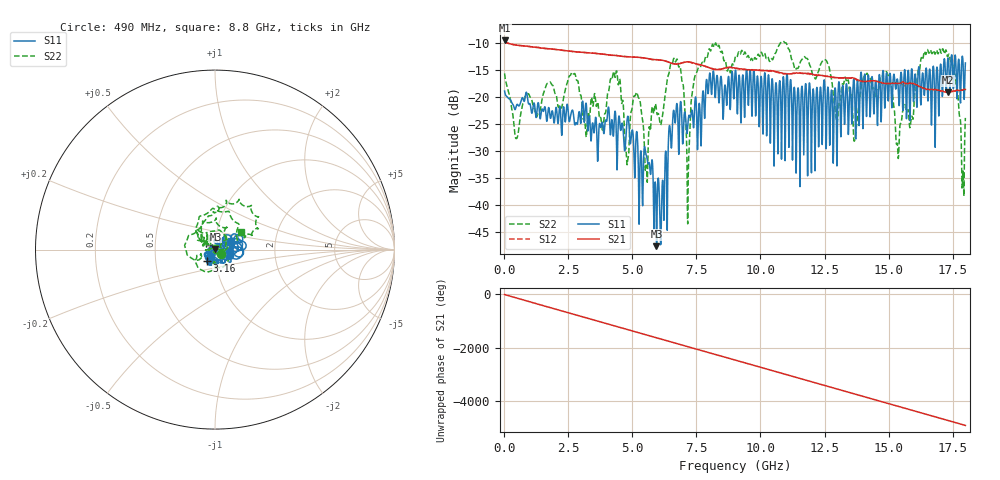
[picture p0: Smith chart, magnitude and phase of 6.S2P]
!Agilent Technologies,E5071C,MY46316741,A.11.02
!Date: Thu Sep 29 15:34:00 2022
!Data & Calibration Information:
!Freq	S11:SOLT2(ON)	S21:SOLT2(ON)	S12:SOLT2(ON)	S22:SOLT2(ON)
!PortZ  Port1:50+j0  Port2:50+j0
!Above PortZ is port z conversion or system Z0 setting when saving the data.
!When reading, reference impedance value at option line is always used.
# Hz S dB R 50
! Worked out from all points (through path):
!   1800 points, 10 MHz to 18 GHz, reference 50 ohm
!   highest |S21| = -9.45 dB at 10 MHz (marker M1); lowest = -19.0 dB at 17.31 GHz (marker M2)
!   group delay of S21, straight-line fit = 756 ps
!   lowest |S11| = -47.6 dB at 5.94 GHz (marker M3), VSWR 1.01, Z = 50.2 + j0.345 ohm
!   |S11| at or under -10 dB: start of sweep to end of sweep
!   |S22| runs from -43.5 to -9.6 dB; largest |S21 - S12| = 0.014
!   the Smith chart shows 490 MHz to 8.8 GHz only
!   S11 on the Smith chart (normalised r, x): 490 MHz: 1.17, -0.07; 3.16 GHz: 0.91, -0.12; 8.8 GHz: 1.19, +0.11
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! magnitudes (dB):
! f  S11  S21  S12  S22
! 10 MHz  -18.8  -9.4  -9.5  -15.6
! 490 MHz  -21.3  -10.3  -10.3  -27.6
! 3.01 GHz  -23.0  -11.6  -11.6  -20.3
! 3.16 GHz  -22.1  -11.7  -11.7  -25.4
! 4.32 GHz  -22.6  -12.2  -12.2  -16.3
! 4.78 GHz  -24.8  -12.5  -12.5  -32.1
! 5.15 GHz  -26.8  -12.6  -12.5  -19.1
! 5.54 GHz  -30.7  -12.7  -12.7  -32.6
! 5.94 GHz  -47.6  -13.0  -13.0  -22.4
! 6.01 GHz  -35.0  -13.0  -13.0  -23.0
! 6.67 GHz  -24.8  -13.8  -13.8  -13.4
! 7.16 GHz  -25.4  -13.4  -13.4  -43.5
! 7.53 GHz  -28.2  -13.8  -13.9  -15.1
! 8.8 GHz  -20.0  -14.4  -14.4  -15.1
! 9.01 GHz  -15.3  -14.6  -14.6  -12.6
! 12.01 GHz  -24.2  -15.6  -15.7  -15.4
! 13.7 GHz  -24.4  -16.5  -16.5  -27.4
! 15.01 GHz  -18.9  -17.4  -17.5  -16.0
! 15.36 GHz  -17.0  -17.4  -17.4  -29.8
! 16.34 GHz  -15.6  -18.3  -18.4  -12.9
! 17.31 GHz  -13.0  -19.0  -19.1  -12.5
! 18 GHz  -13.6  -18.5  -18.6  -23.8
